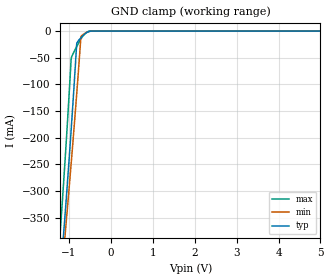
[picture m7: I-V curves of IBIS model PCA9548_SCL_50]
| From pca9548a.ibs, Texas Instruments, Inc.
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[Model]   PCA9548_SCL_50
Model_type  Terminator
| variable   typ   min   max
C_comp   7.66pF   5.67pF   11.33pF
| C_tri-state   7.66pF   5.67pF   11.33pF
[Temperature Range]   40   100   -40
| Ambient temperature   25   85   -40
[Voltage range]   5   4.5   5.5
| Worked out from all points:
|   GND clamp passes 1 mA (typ) near -0.53 V on its own axis
[GND Clamp]
| PCA9548_SCL_50
|   Voltage   I(typ)   I(min)   I(max)
-5.5V     -3.656A    -3.511A    -3.814A
-1.215V   -469.9mA   -491.5mA   -387.7mA
-1.17V    -425.8mA   -453mA     -337mA
-1.125V   -380.5mA   -413.8mA   -284.5mA
-1.1V     -354.8mA   -391.7mA   -254.5mA
-1.075V   -328.7mA   -369.3mA   -223.8mA
-1.005V   -253.3mA   -305.4mA   -134.2mA
-945mV    -185.6mA   -249mA     -52.16mA
-810mV    -22.62mA   -115.3mA   -28.77mA
-710mV    -12.38mA   -10.09mA   -14.56mA
-560mV    -2.241mA   -2.075mA   -1.504mA
5V        452.7pA    1.006nA    296.3pA
